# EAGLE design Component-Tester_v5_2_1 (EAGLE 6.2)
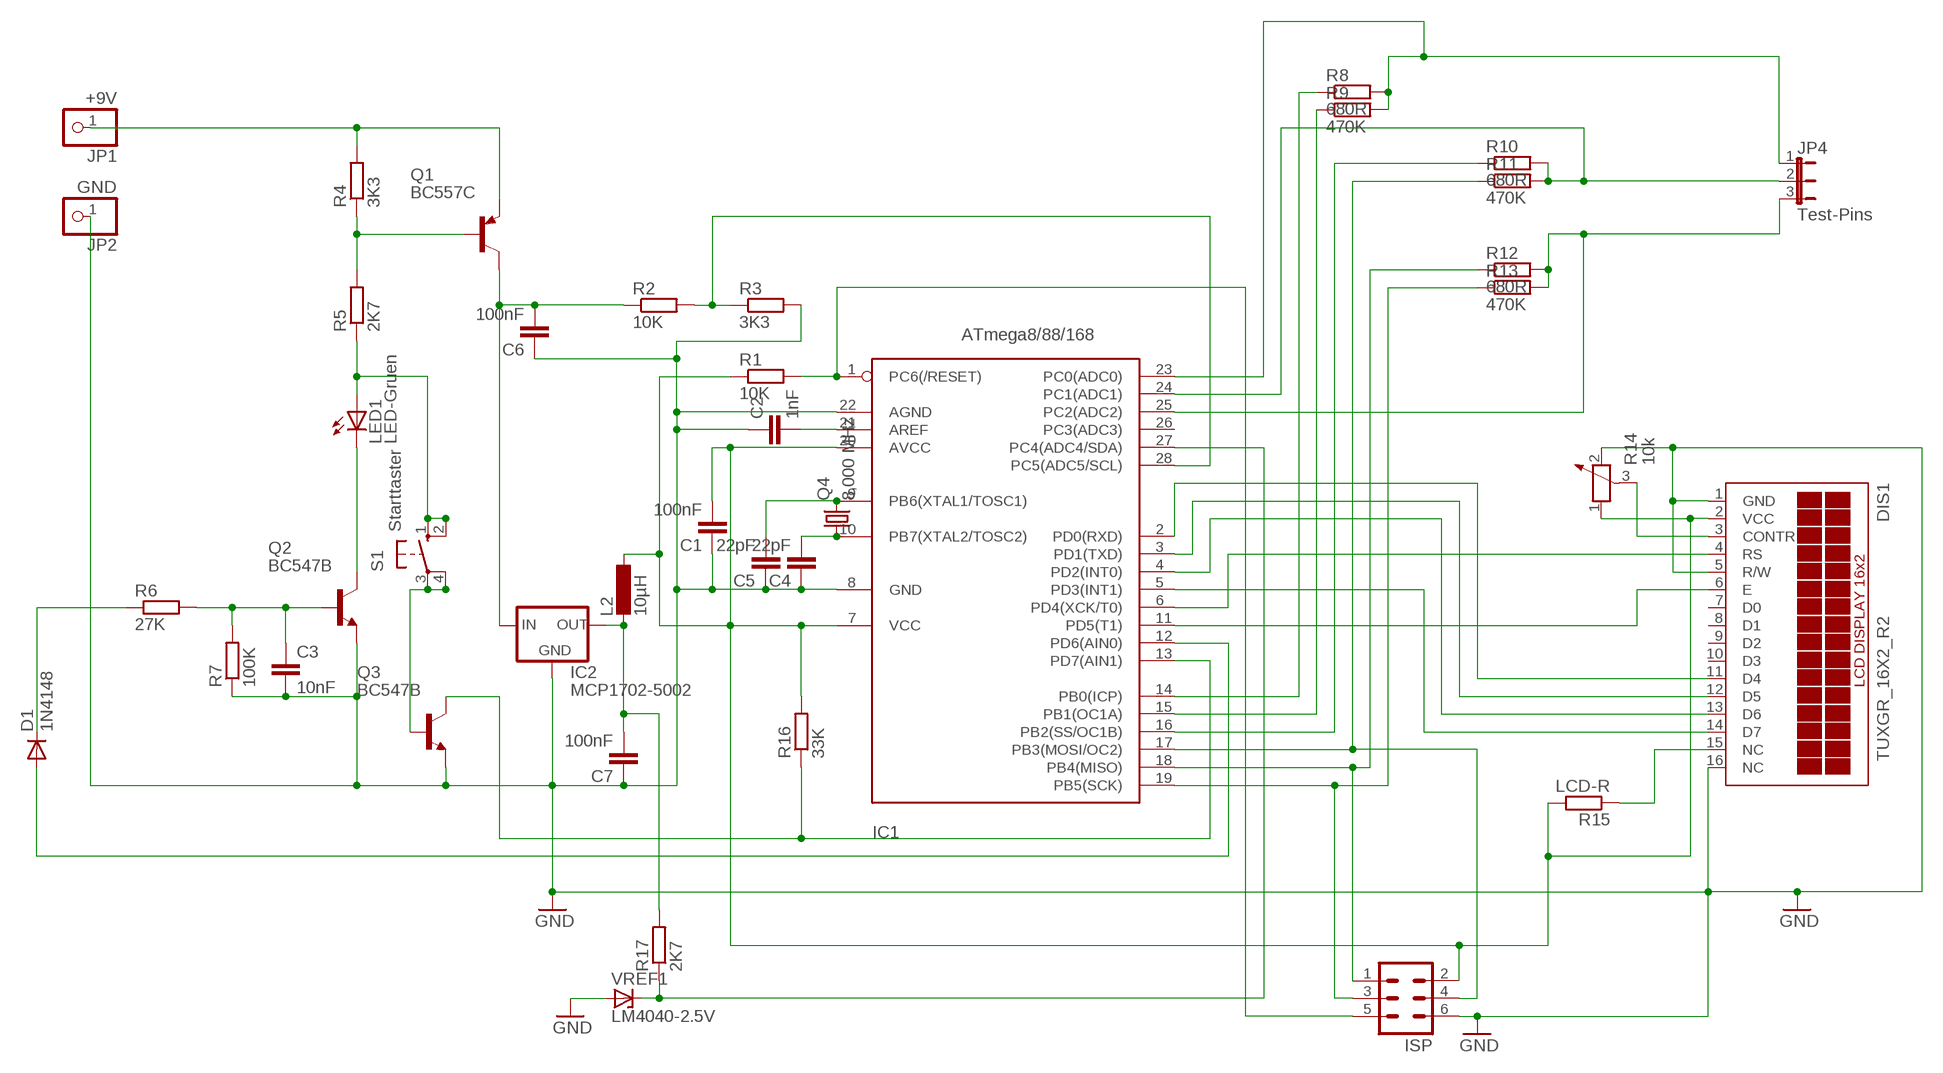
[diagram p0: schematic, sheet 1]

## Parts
C1  100nF  C5/3.5  [C5B3.5]
C2  1nF  C2.5/2  [C2.5-2]
C3  10nF  C5/3.5  [C5B3.5]
C4  22pF  C-EU025-025X050  [C025-025X050]
C5  22pF  C-EU025-025X050  [C025-025X050]
C6  100nF  C5/3.5  [C5B3.5]
C7  100nF  C5/3.5  [C5B3.5]
D1  1N4148  1N4148DO35-7  [DO35-7]
DIS1  TUXGR_16X2_R2  [TUXGR_16X2_R2]
IC1  ATmega8/88/168  MEGA8-P  [DIL28-3]
IC2  MCP1702-5002  [TO92-LOWDROP]
ISP  ML6L  [ML6L]
JP1  +9V  PINHD-1X1  [1X01]
JP2  GND  PINHD-1X1  [1X01]
JP4  Test-Pins  JP2E  [JP2]
L2  10µH  L-EU0207/10  [0207/10]
LED1  LED-Gruen  LED5MM  [LED5MM]
Q1  BC557C  [TO92-EBC]
Q2  BC547B  [TO92]
Q3  BC547B  [TO92]
Q4  8,000 MHz  CRYSTALHC49S  [HC49/S]
R1  10K  R-EU_0207/10  [0207/10]
R2  10K  R-EU_0207/10  [0207/10]
R3  3K3  R-EU_0207/10  [0207/10]
R4  3K3  R-EU_0207/10  [0207/10]
R5  2K7  R-EU_0207/10  [0207/10]
R6  27K  R-EU_0207/10  [0207/10]
R7  100K  R-EU_0207/10  [0207/10]
R8  680R  R-EU_0207/10  [0207/10]
R9  470K  R-EU_0207/10  [0207/10]
R10  680R  R-EU_0207/10  [0207/10]
R11  470K  R-EU_0207/10  [0207/10]
R12  680R  R-EU_0207/10  [0207/10]
R13  470K  R-EU_0207/10  [0207/10]
R14  10k  POTENTIOMETER_PT-10  [PT-10]
R15  LCD-R  R-EU_0207/10  [0207/10]
R16  33K  R-EU_0207/10  [0207/10]
R17  2K7  R-EU_0207/10  [0207/10]
S1  Starttaster  10-XX  [B3F-10XX]
VREF1  LM4040-2.5V  LM4040  [TO92-VREF]

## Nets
GND: C1.1 C2.1 C3.2 C4.1 C5.1 C6.1 C7.1 DIS1.1(GND) DIS1.5(R/W) DIS1.16(NC) IC1.8(GND) IC1.22(AGND) IC2.GND ISP.6 JP2.1 Q2.1(E) Q3.1(E) R3.2 R7.1 R14.2 VREF1.-
N$2: C6.2 IC2.IN Q1.C R2.1
N$3: IC1.1(PC6(/RESET)) ISP.5 R1.2
N$4: C2.2 IC1.21(AREF)
N$5: Q1.B R4.1 R5.2
N$6: IC1.28(PC5(ADC5/SCL)) R2.2 R3.1
N$8: C1.2 DIS1.2(VCC) IC1.7(VCC) IC1.20(AVCC) ISP.2 L2.1 R1.1 R14.1 R15.2 R16.2
N$9: LED1.K(C) Q2.3(C)
N$10: IC1.13(PD7(AIN1)) Q3.3(C) R16.1
N$11: C3.1 Q2.2(B) R6.2 R7.2
N$12: D1.A IC1.12(PD6(AIN0))
N$13: IC1.25(PC2(ADC2)) JP4.3 R12.2 R13.2
N$14: Q3.2(B) S1.3(P) S1.4(P1)
N$15: IC1.24(PC1(ADC1)) JP4.2 R10.2 R11.2
N$16: IC1.23(PC0(ADC0)) JP4.1 R8.2 R9.2
N$17: C7.2 IC2.OUT L2.2 R17.2
N$18: IC1.18(PB4(MISO)) ISP.1 R12.1
N$19: IC1.14(PB0(ICP)) R8.1
N$20: IC1.15(PB1(OC1A)) R9.1
N$21: IC1.16(PB2(SS/OC1B)) R10.1
N$22: IC1.19(PB5(SCK)) ISP.3 R13.1
N$23: LED1.A R5.1 S1.1(S) S1.2(S1)
N$24: DIS1.3(CONTR) R14.3
N$25: DIS1.4(RS) IC1.6(PD4(XCK/T0))
N$26: DIS1.6(E) IC1.11(PD5(T1))
N$27: DIS1.11(D4) IC1.2(PD0(RXD))
N$28: DIS1.12(D5) IC1.3(PD1(TXD))
N$29: DIS1.13(D6) IC1.4(PD2(INT0))
N$30: DIS1.14(D7) IC1.5(PD3(INT1))
N$31: C4.2 IC1.10(PB7(XTAL2/TOSC2)) Q4.1
N$32: DIS1.15(NC) R15.1
N$33: JP1.1 Q1.E R4.2
N$34: C5.2 IC1.9(PB6(XTAL1/TOSC1)) Q4.2
N$37: D1.C R6.1
N$39: IC1.17(PB3(MOSI/OC2)) ISP.4 R11.1
N$40: IC1.27(PC4(ADC4/SDA)) R17.1 VREF1.+
Unconnected: DIS1.7(D0) DIS1.8(D1) DIS1.9(D2) DIS1.10(D3) IC1.26(PC3(ADC3))

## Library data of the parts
C1-C3 C6 C7 = capacitor-wima:C: CAPACITOR
C4 C5 = rcl:C-EU: CAPACITOR, European symbol
D1 = diode:1N4148: DIODE
DIS1 = display-lcd:TUXGR_16X2_R2: Tuxgraphics LCD display 16x2 characters reflective, without background light Source: tuxgr_12x2_r2.pdf; OC_FARNELL: unknown; OC_NEWARK: unknown
IC1 = avr-6:MEGA8-P: MICROCONTROLLER 8 Kbytes FLASH 1 kbytes SRAM 512 bytes EEPROM USART 4-channel 10 bit ADC 2-channel 8 bit ADC
IC2 = asko:MCP1702-5002
ISP = con-ml:ML6L: HARTING; OC_FARNELL: unknown; OC_NEWARK: unknown
JP1 JP2 = pinhead:PINHD-1X1: PIN HEADER
JP4 = jumper:JP2E: JUMPER
L2 = rcl:L-EU: INDUCTOR, European symbol
LED1 = led:LED: LED
Q1 = transistor-pnp:BC557*: PNP Transistror
Q2 Q3 = transistor-npn:BC547*: NPN Transistor
Q4 = crystal:CRYSTAL: CRYSTAL; OC_FARNELL: 1667008; OC_NEWARK: unknown
R1-R13 R15-R17 = resistor:R-EU_: RESISTOR, European symbol
R14 = rcl:POTENTIOMETER_: Potentiometer
S1 = switch-omron:10-XX: OMRON SWITCH; MPN: B3F-1000; OC_FARNELL: 176432; OC_NEWARK: 36M3542
VREF1 = asko:LM4040

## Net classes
0 default: width 0.406 mm, drill 0.8 mm

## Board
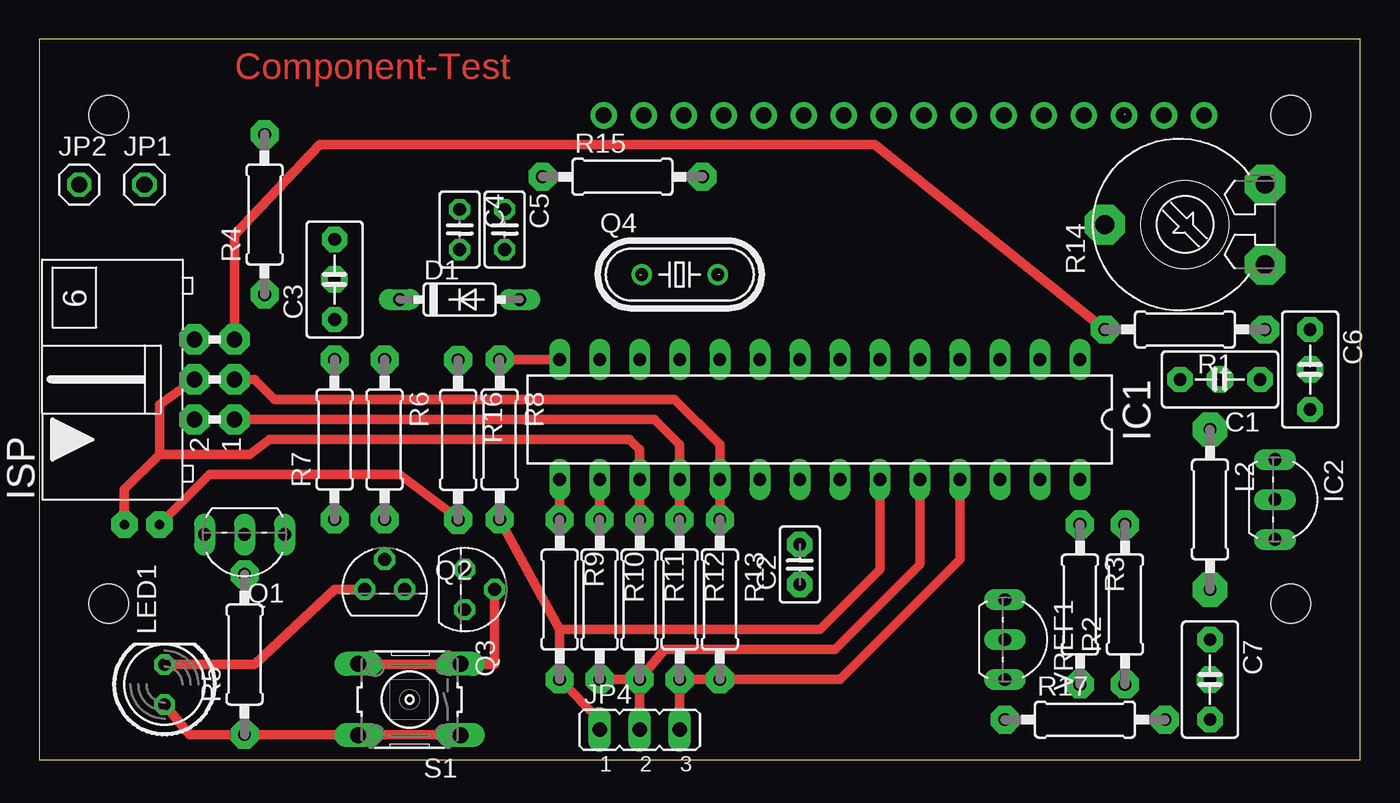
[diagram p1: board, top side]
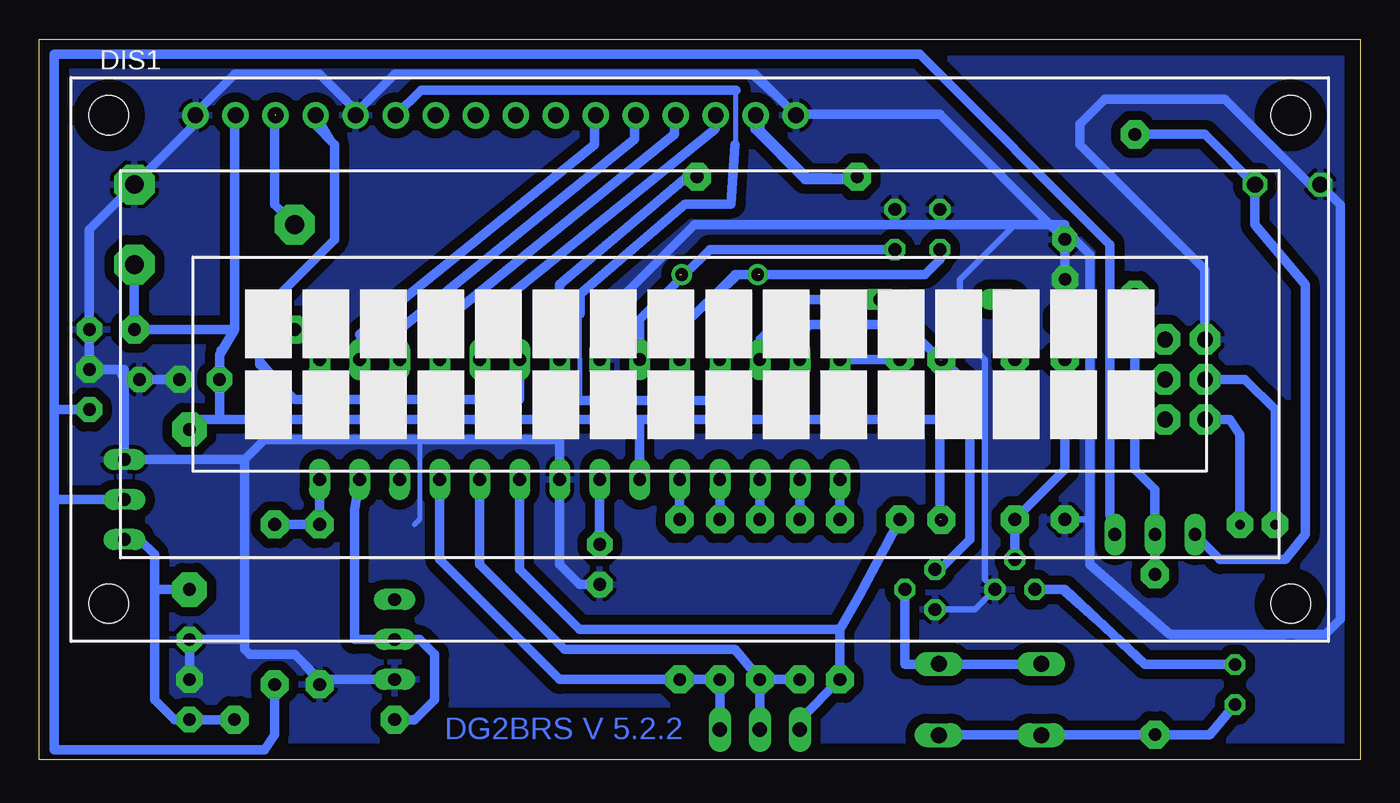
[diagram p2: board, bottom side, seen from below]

Size 83.82 x 45.72 mm. Coordinates in mm from the lower left corner, seen from the top.
Outline: 0,0 83.82,0 83.82,45.72 0,45.72 0,0
Copper layers (1*16): Top 0.035mm / dielectric 1.5mm / Bottom 0.035mm
Design rules: minimum track width 10mil, minimum drill 24mil, track to track 8mil, track to pad 8mil, pad to pad 8mil, via to via 8mil, smd to smd 8mil, copper to edge 40mil, drill to drill 8mil, minimum pad ring 10mil, minimum via ring 8mil, stop-mask expansion 4mil, vias tented up to drill 0mil, thermal gap 10mil

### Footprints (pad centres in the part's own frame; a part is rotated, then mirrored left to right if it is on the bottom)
C5B3.5 = drill 0.813 pad 1.6 octagon: 1 -2.54,0; 2 2.54,0
C2.5-2 = drill 0.813 pad 1.6 octagon: 1 -1.27,0; 2 1.27,0
C025-025X050 = drill 0.813 octagon: 1 -1.27,0; 2 1.27,0
DO35-7 = drill 0.813 long: A 3.81,0; C -3.81,0
TUXGR_16X2_R2 = drill 1 pad 1.676: 1 -32,15.5; 2 -29.46,15.5; 3 -26.92,15.5; 4 -24.38,15.5; 5 -21.84,15.5; 6 -19.3,15.5; 7 -16.76,15.5; 8 -14.22,15.5; 9 -11.68,15.5; 10 -9.14,15.5; 11 -6.6,15.5; 12 -4.06,15.5; 13 -1.52,15.5; 14 1.02,15.5; 15 3.56,15.5; 16 6.1,15.5 | hole 2.5: -37.5,-15.5; 37.5,-15.5; -37.5,15.5; 37.5,15.5
DIL28-3 = drill 0.813 long: 1 -16.51,-3.81; 2 -13.97,-3.81; 3 -11.43,-3.81; 4 -8.89,-3.81; 5 -6.35,-3.81; 6 -3.81,-3.81; 7 -1.27,-3.81; 8 1.27,-3.81; 9 3.81,-3.81; 10 6.35,-3.81; 11 8.89,-3.81; 12 11.43,-3.81; 13 13.97,-3.81; 14 16.51,-3.81; 15 16.51,3.81; 16 13.97,3.81; 17 11.43,3.81; 18 8.89,3.81; 19 6.35,3.81; 20 3.81,3.81; 21 1.27,3.81; 22 -1.27,3.81; 23 -3.81,3.81; 24 -6.35,3.81; 25 -8.89,3.81; 26 -11.43,3.81; 27 -13.97,3.81; 28 -16.51,3.81
TO92-LOWDROP = drill 0.813 long: GND -3.81,0; IN -1.27,0; OUT 1.27,0
ML6L = drill 1 pad 1.93 octagon: 1 -2.54,-1.27; 2 -2.54,1.27; 3 0,-1.27; 4 0,1.27; 5 2.54,-1.27; 6 2.54,1.27
1X01 = drill 1.016 octagon: 1 0,0
JP2 = drill 0.914 long: 1 -2.54,0; 2 0,0; 3 2.54,0
0207/10 = drill 0.813 pad 2.184 octagon: 1 -5.08,0; 2 5.08,0
LED5MM = drill 0.813 octagon: A -1.27,0; K 1.27,0
TO92-EBC = drill 0.813 long: B 0,-1.27; C -2.54,-1.27; E 2.54,-1.27
TO92 = drill 0.813 octagon: 1 1.27,0; 2 0,1.905; 3 -1.27,0
HC49/S = drill 0.813: 1 -2.413,0; 2 2.413,0
0207/10' = drill 0.813 pad 1.778 octagon: 1 -5.08,0; 2 5.08,0
PT-10 = drill 1.2 pad 2.54 octagon: 1 -2.54,-5.08; 2 2.54,-5.08; 3 0,5.08
B3F-10XX = drill 1.016 long: 1 -3.251,2.261; 2 3.251,2.261; 3 -3.251,-2.261; 4 3.251,-2.261
TO92-VREF = drill 0.813 long: + 0,0; - 2.54,0; NC -2.54,0

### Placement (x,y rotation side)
C1  74.93,24.13 180 top
C2  48.26,12.38 90 top
C3  18.73,30.48 90 top
C4  26.67,33.66 270 top
C5  29.53,33.66 270 top
C6  80.64,24.77 270 top
C7  74.3,5.08 270 top
D1  26.67,29.21 0 top
DIS1  41.91,25.4 0 bottom
IC1  49.53,21.59 180 top
IC2  78.42,15.24 270 top
ISP  11.11,24.13 90 top
JP1  6.67,36.51 0 top
JP2  2.54,36.51 0 top
JP4  38.1,1.91 0 top
L2  74.3,15.88 270 top
LED1  7.94,4.76 90 top
Q1  13.02,13.02 180 top
Q2  21.91,10.79 0 top
Q3  26.99,10.79 270 top
Q4  40.64,30.8 0 top
R1  10K  [0207/10']  72.71,27.3 180 top
R2  10K  [0207/10']  68.9,9.84 90 top
R3  3K3  [0207/10']  66.04,9.84 270 top
R4  3K3  [0207/10']  14.29,34.61 90 top
R5  2K7  [0207/10']  13.02,6.67 90 top
R6  27K  [0207/10']  21.91,20.32 270 top
R7  100K  [0207/10']  18.73,20.32 90 top
R8  680R  [0207/10']  29.21,20.32 270 top
R9  470K  [0207/10']  33.02,10.16 270 top
R10  680R  [0207/10']  35.56,10.16 270 top
R11  470K  [0207/10']  38.1,10.16 270 top
R12  680R  [0207/10']  40.64,10.16 270 top
R13  470K  [0207/10']  43.18,10.16 270 top
R14  72.71,33.97 90 top
R15  LCD-R  [0207/10']  37,37 0 top
R16  33K  [0207/10']  26.57,20.3 270 top
R17  2K7  [0207/10']  66.36,2.54 0 top
S1  23.5,3.81 180 top
VREF1  61.28,7.62 270 top

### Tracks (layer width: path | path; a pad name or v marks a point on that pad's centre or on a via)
GND  (via drill 0.8 pad 1.68)
  Bottom 0.305: 59.69,20.32 59.69,15.24 60.01,14.92
  Bottom 0.406: 60.96,43.5 38.73,43.5 35.56,40.64 DIS1.16 | 67.63,6.67 R3.2 | 19.05,15.24 R7.1 17.14,15.24 | Q3.1 24.45,9.53 Q2.1 23.81,11.43 23.81,25.4 25.4,26.99 25.4,30.48 21.91,33.97
  Bottom 0.61: 78.74,24.77 v80.64,24.77 C6.1 80.64,33.66 R14.2 73.98,40.32 73.98,40.96 71.44,43.5 66.04,43.5 63.82,41.27 63.82,40.96 61.28,43.5 38.42,43.5 35.88,40.96 26.67,40.96 C3.2 | 78.74,24.77 78.42,24.13 | 78.42,24.13 C1.1 v74.93,24.13 | 78.42,24.13 78.42,19.68 79.06,19.05 IC2.GND 70.8,19.05 | 70.8,7.62 70.8,6.99 70.48,6.67 67.63,6.67 66.04,5.08 R3.2 65.72,5.08 VREF1.- | 70.8,7.62 70.8,19.05 | 70.8,7.62 C7.1 v74.3,5.08 | 70.8,19.05 69.53,20.32 59.69,20.32 50.8,20.32 IC1.22 50.8,12.38 49.53,11.11 C2.1 | IC1.8 48.26,27.94 42.23,33.97 29.53,33.97 | 29.53,33.97 26.67,33.97 | 26.67,33.97 21.91,33.97 18.73,33.97 C3.2 | C3.2 18.1,33.02 17.14,32.07 17.14,15.24 17.14,12.38 12.06,7.94 2.22,7.94 1.27,8.89 1.27,35.24 JP2.1 3.17,36.51 8.57,41.91 16.19,41.91 17.78,40.32 17.78,39.05 9.84,31.11 ISP.6 | C4.1 26.67,33.97 | C5.1 29.53,33.97 | C3.2 v18.73,30.48 | 78.42,24.13 78.42,24.77 78.74,24.77
  pour Bottom (isolate 0.61): -0.32,46.04 84.14,46.04 84.14,-0.32 -0.32,-0.32
N$1  (via drill 0.8)
  other vias: 4.45,40.96
N$2
  Bottom 0.406: Q1.C 15.88,15.24 15.88,32.7
  Bottom 0.61: 82.87,22.23 82.87,44.77 27.94,44.77 15.88,32.7 15.88,15.56 Q1.C | 82.87,16.51 82.87,0.64 69.53,0.64 68.9,1.59 R2.1 | 82.87,22.23 C6.2 | 82.87,22.23 82.87,16.51 | 82.87,16.51 IC2.IN
N$3
  Top 0.61: R1.2 53.02,39.05 17.78,39.05 12.38,33.34 ISP.5
  Bottom 0.406: IC1.1 R1.2
  Bottom 0.61: IC1.1 66.04,25.72 R1.2
N$4
  Bottom 0.61: IC1.21 C2.2
N$5
  Bottom 0.61: R4.1 14.29,18.41 13.02,17.14 Q1.B R5.2
N$6
  Bottom 0.61: IC1.28 R3.1 R2.2
N$7  (via drill 0.8)
  other vias: 4.45,9.84
N$8  (via drill 0.6 pad 1.68)  (2 unrouted)
  Top 0.61: 26.67,15.24 22.86,18.1 10.79,18.1 v7.62,14.92
  Bottom 0.406: 71.44,27.3 71.44,40.64 DIS1.2 | 42.62,37.08 R15.2 | 72.39,25.72 72.39,26.04 | R14.1 77.79,31.75
  Bottom 0.61: 42.62,37.08 50.8,30.16 IC1.7 50.8,21.59 | 45.72,21.59 IC1.20 | 26.67,15.24 26.67,21.59 45.72,21.59 | 45.72,21.59 50.8,21.59 | 50.8,21.59 72.39,21.59 | 72.39,21.59 73.66,21.59 L2.1 | 72.39,21.59 C1.2 72.39,25.72 71.44,27.3 | 71.44,27.3 71.44,40.96 | R14.1 R1.1 71.44,27.3 | ISP.2 8.26,21.59 7.62,20.64 v7.62,14.92
N$9
  Top 0.61: Q2.3 18.73,10.79 13.65,6.03 LED1.K
  Bottom 0.406: 13.65,6.03 19.05,10.79 Q2.3
  Bottom 0.61: Q2.3 18.73,10.79 13.65,6.03 LED1.K
N$10  (1 unrouted)
  Bottom 0.61: Q3.3 26.67,12.06 24.77,13.97 24.77,23.81 26.67,25.4 28.89,27.62 34.92,27.62 35.56,26.99 IC1.13
N$11
  Bottom 0.406: C3.1 R7.2 18.73,18.41
  Bottom 0.61: Q2.2 R6.2 18.73,18.41 C3.1
N$12
  Bottom 0.61: D1.A 35.56,29.21 38.1,26.67 IC1.12
N$13
  Top 0.406: IC1.25 58.42,13.97
  Top 0.61: JP4.3 R12.2 R13.2 50.8,5.08 58.42,12.7 IC1.25
  Bottom 0.61: JP4.3 R12.2 R13.2 50.8,5.08 58.42,12.7 IC1.25
N$14
  Top 0.61: Q3.2 28.89,6.03 20.32,6.03
  Bottom 0.406: 28.89,6.03 S1.4 20.64,6.03 20.32,6.03 20,6.03 S1.3
  Bottom 0.61: 20.32,6.03 28.89,6.03 Q3.2
N$15
  Top 0.406: IC1.24 55.88,13.34
  Top 0.61: R10.2 R11.2 | R11.2 JP4.2 | R11.2 39.69,6.99 50.48,6.99 55.88,12.38 IC1.24
  Bottom 0.61: R10.2 R11.2 | R11.2 JP4.2 | R11.2 39.69,6.99 50.48,6.99 55.88,12.38 IC1.24
N$16
  Top 0.406: 35.56,2.54 JP4.1
  Top 0.61: 35.56,2.54 R9.2 33.02,8.26 | R8.2 33.02,8.26 | 33.02,8.26 49.53,8.26 53.34,12.06 IC1.23
  Bottom 0.406: 33.02,8.26 R8.2
  Bottom 0.61: 33.02,8.26 49.53,8.26 53.34,12.06 IC1.23 | JP4.1 35.56,2.54 R9.2 33.02,8.26 | 33.02,8.26 31.75,10.48 R8.2
N$17
  Bottom 0.61: 76.52,10.79 76.52,3.81 75.25,2.54 C7.2 R17.2 | IC2.OUT 77.47,13.97 76.52,13.02 76.52,10.79 | 76.52,10.79 L2.2
N$18
  Top 0.61: R12.1 IC1.18 40.64,20 39.05,21.59 ISP.1
  Bottom 0.61: IC1.18 R12.1
N$19
  Top 0.61: IC1.14 R8.1
  Bottom 0.61: IC1.14 R8.1
N$20
  Top 0.61: IC1.15 R9.1
  Bottom 0.61: IC1.15 R9.1
N$21
  Top 0.61: IC1.16 R10.1
  Bottom 0.61: IC1.16 R10.1
N$22
  Top 0.61: R13.1 IC1.19 43.18,20 40.32,22.86 14.92,22.86 13.65,24.13 ISP.3
  Bottom 0.61: IC1.19 R13.1
N$23
  Top 0.61: 26.67,1.59 R5.1 9.53,1.59 LED1.A
  Bottom 0.406: 16.51,1.59 R5.1 9.53,1.59 | 16.51,1.59 21.27,1.59 S1.2 | S1.1 16.51,1.59
  Bottom 0.61: 26.67,1.59 9.53,1.59 LED1.A
N$24  (1 unrouted)
  Bottom 0.61: R14.3 68.9,35.24 68.9,40.96
N$25
  Bottom 0.406: 67.63,22.86 69.85,25.4 69.85,28.26 69.85,28.57 | 65.09,39.05 66.04,40.64 DIS1.4
  Bottom 0.61: 66.36,40.96 66.36,40.32 65.09,39.05 65.09,33.02 69.85,28.26 69.85,25.08 67.63,22.86 53.34,22.86 IC1.6
N$26
  Bottom 0.305: 49.5,22.8 49.53,28.26 | 39.6,39.14 39.6,42.5
  Bottom 0.406: 40.64,23.86 IC1.11 | 49.53,28.26 49.5,28.29 | 39.69,39.05 39.6,39.14
  Bottom 0.61: 40.64,23.86 40.75,22.8 49.5,22.8 | 49.5,28.29 49.5,29.57 42.84,35.27 39.92,35.27 39.69,39.05 | 39.6,42.5 59.61,42.5 DIS1.6 | IC1.11 40.64,22.86
N$27
  Bottom 0.406: 63.5,26.99 IC1.2 | DIS1.11 48.58,39.05
  Bottom 0.61: 63.5,26.99 48.58,39.05 48.58,40.96
N$28
  Bottom 0.406: DIS1.12 46.04,39.37
  Bottom 0.61: IC1.3 60.96,27.3 46.04,39.37 46.04,40.96
N$29
  Bottom 0.406: DIS1.13 43.5,39.69
  Bottom 0.61: IC1.4 58.42,27.62 43.5,39.69 43.5,40.96
N$30
  Bottom 0.406: DIS1.14 40.96,40.01
  Bottom 0.61: IC1.5 55.88,27.94 40.96,40.01 40.96,40.96
N$31  (1 unrouted)
  Bottom 0.406: 43.18,27.3 39.69,30.48 39.37,30.8
  Bottom 0.61: C4.2 26.67,31.75 27.62,30.8 38.1,30.8 39.37,30.8 39.69,30.8 43.18,27.3 IC1.10
N$32
  Bottom 0.406: R15.1 35.08,37.08 38,40 38,40.55 DIS1.15
N$33
  Bottom 0.61: R4.2 9.84,39.69 JP1.1 6.67,33.97 3.49,30.16 3.49,14.29 4.76,12.7 8.89,12.7 Q1.E
N$34  (1 unrouted)
  Bottom 0.61: C5.2 41.27,32.38 42.86,30.8 | 42.86,30.8 45.72,27.94 IC1.9 | 43.18,30.8 42.86,30.8
N$35  (via drill 0.8)
  other vias: 79.38,9.84
N$36  (via drill 0.8)
  other vias: 79.38,40.96
N$37
  Bottom 0.406: D1.C 21.91,28.57 R6.1
  Bottom 0.61: R6.1 21.91,28.26 D1.C
N$38
  Bottom 0.61: 31.75,36.83 35.24,36.83 38.42,40.01 38.42,40.96
N$39  (via drill 0.6 pad 1.68)
  Top 0.61: R11.1 IC1.17 38.1,19.68 37.47,20.32 14.61,20.32 13.34,19.37 7.62,19.37 | 7.62,19.37 7.62,22.54 ISP.4 | 7.62,19.37 5.4,17.14 v5.4,14.92
  Bottom 0.61: IC1.17 R11.1 | ISP.4 7.3,24.13 5.4,22.23 v5.4,14.92
N$40
  Bottom 0.61: IC1.27 63.82,15.88 63.82,7.62 VREF1.+ 59.69,7.62 58.74,6.67 58.74,3.81 60.01,2.54 R17.1

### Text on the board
Top: Component-Test
Bottom: DG2BRS V 5.2.2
